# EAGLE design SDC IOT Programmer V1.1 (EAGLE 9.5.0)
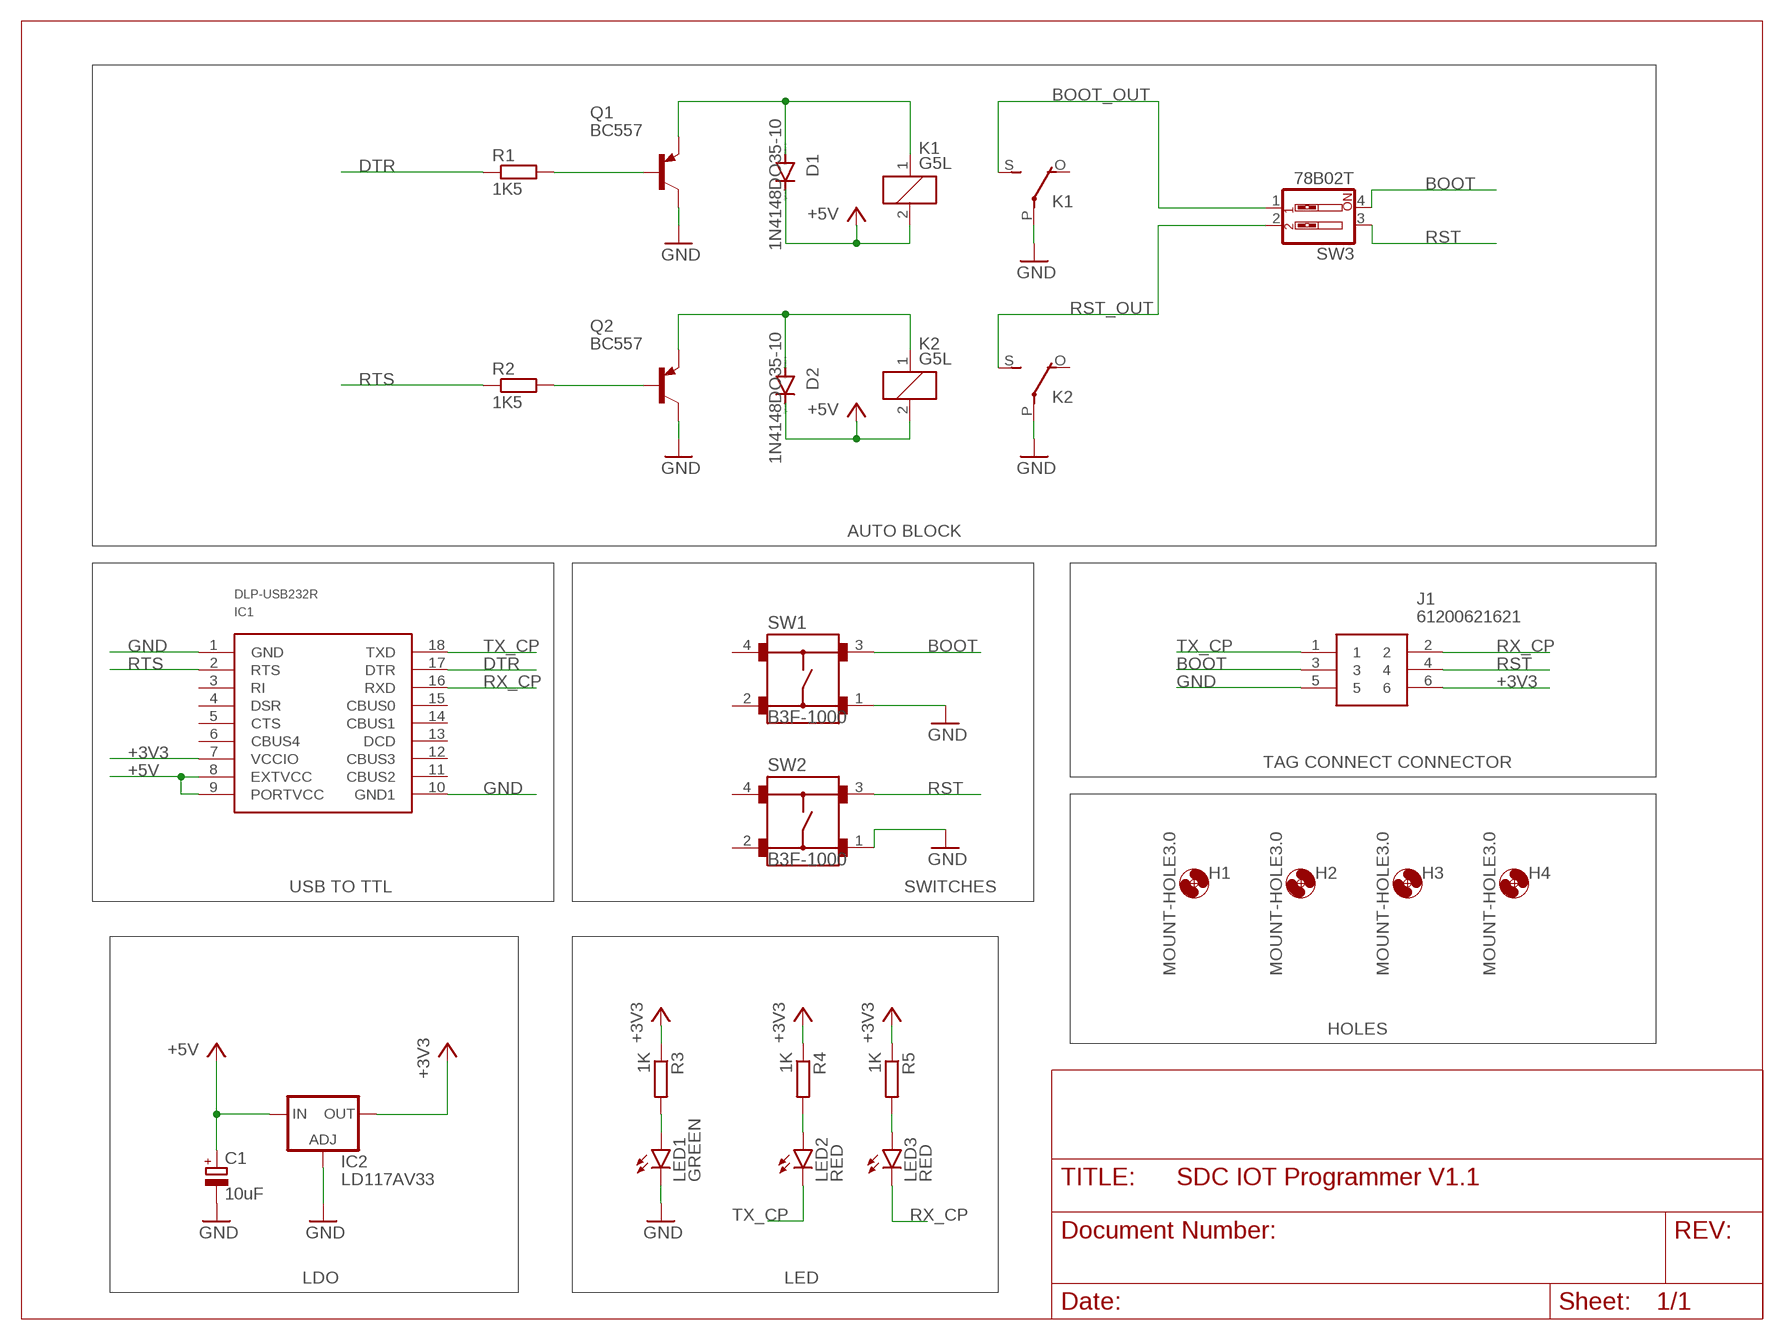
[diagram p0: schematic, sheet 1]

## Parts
C1  10uF  CPOL-EUE2.5-5  [E2,5-5]
D1  1N4148DO35-10  [DO35-10]
D2  1N4148DO35-10  [DO35-10]
H1  MOUNT-HOLE3.0  [3,0]
H2  MOUNT-HOLE3.0  [3,0]
H3  MOUNT-HOLE3.0  [3,0]
H4  MOUNT-HOLE3.0  [3,0]
IC1  DLP-USB232R  [DLP-USB232R]
IC2  LD117AV33  [TO220L1]
J1  61200621621  [SHDR6W64P254_2X3_1528X910X910P]
K1  G5L  [G5LE]
K2  G5L  [G5LE]
LED1  GREEN  LED3MM  [LED3MM]
LED2  RED  LED3MM  [LED3MM]
LED3  RED  LED3MM  [LED3MM]
Q1  BC557  [TO92-EBC]
Q2  BC557  [TO92-EBC]
R1  1K5  R-EU_0207/10  [0207/10]
R2  1K5  R-EU_0207/10  [0207/10]
R3  1K  R-EU_0207/10  [0207/10]
R4  1K  R-EU_0207/10  [0207/10]
R5  1K  R-EU_0207/10  [0207/10]
SW1  B3F-1000  [B3F-1000]
SW2  B3F-1000  [B3F-1000]
SW3  78B02T  SW_DIP-2  [EDG-02]

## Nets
+3V3: IC1.7(VCCIO) IC2.2(OUT) J1.6 R3.1 R4.1 R5.1
+5V: C1.+ D1.C D2.C IC1.8(EXTVCC) IC1.9(PORTVCC) IC2.3(IN) K1.2 K2.2
BOOT: J1.3 SW1.3 SW3.4
BOOT_OUT: K1.S(2:S) SW3.1
DTR: IC1.17(DTR) R1.1
GND: C1.- IC1.1(GND) IC1.10(GND1) IC2.1(ADJ) J1.5 K1.P(2:P) K2.P(2:P) LED1.K(C) Q1.C Q2.C SW1.1 SW2.1
N$7: LED2.A R4.2
N$12: Q1.B R1.2
N$13: Q2.B R2.2
N$14: D1.A K1.1 Q1.E
N$15: D2.A K2.1 Q2.E
N$16: LED1.A R3.2
N$17: LED3.A R5.2
RST: J1.4 SW2.3 SW3.3
RST_OUT: K2.S(2:S) SW3.2
RTS: IC1.2(RTS) R2.1
RX_CP: IC1.16(RXD) J1.2 LED3.K(C)
TX_CP: IC1.18(TXD) J1.1 LED2.K(C)
Unconnected: IC1.3(RI) IC1.4(DSR) IC1.5(CTS) IC1.6(CBUS4) IC1.11(CBUS2) IC1.12(CBUS3) IC1.13(DCD) IC1.14(CBUS1) IC1.15(CBUS0) K1.O(2:O) K2.O(2:O) SW1.2 SW1.4 SW2.2 SW2.4

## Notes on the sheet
- AUTO BLOCK
- TAG CONNECT CONNECTOR
- USB TO TTL | SWITCHES
- HOLES
- LDO | LED

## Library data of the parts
C1 = rcl:CPOL-EU: POLARIZED CAPACITOR, European symbol; SPICEPREFIX: C
D1 D2 = diode:1N4148: DIODE
H1-H4 = holes:MOUNT-HOLE: MOUNTING HOLE with drill center marker
IC1 = USB232:DLP-USB232R
IC2 = v-reg:LD117A?*: Low drop fixed and adjustable positive voltage regulators 1 A Source: http://www.st.com/stonline/products/literature/ds/7194/ld1117axx.pdf
J1 = MOLEX:61200621621: Wurth Elektronik PCB Header WR-BHD, 6 Way, 2.54mm Pitch, 2 Row, Straight, Through Hole Source: Datasheet; DESCRIPTION: Wurth Elektronik PCB Header WR-BHD, 6 Way, 2.54mm Pitch, 2 Row, Straight, Through Hole; HEIGHT: 9.1mm; MANUFACTURER_NAME: Wurth Elektronik; MANUFACTURER_PART_NUMBER: 61200621621; MOUSER_PART_NUMBER: 710-61200621621; MOUSER_PRICE-STOCK: https://www.mouser.co.uk/ProductDetail/Wurth-Elektronik/61200621621?qs=PhR8RmCirEbjX8n1RKw4Jw%3D%3D
K1 K2 = relay:G5L: RELAY 1 x switch, 10 A/120 V AC, 8 A/30 V ADC, Omron; OC_FARNELL: unknown; OC_NEWARK: unknown
LED1-LED3 = led:LED: LED
Q1 Q2 = transistor-pnp:BC557*: PNP Transistror
R1-R5 = rcl:R-EU_: RESISTOR, European symbol; SPICEPREFIX: R
SW1 SW2 = Switch:B3F-1000: Tactile Switch SPST-NO Top Actuated Through Hole Manufacturer's datasheet; CREATED_BY: PCBLayout.com; DIGI_KEY_PART_NUMBER: SW400-ND; MANUFACTURER: Omron Electronics Inc-EMC Div; MPN: B3F-1000; PACKAGE: SPST-NO
SW3 = special:SW_DIP-2: DIP SWITCH

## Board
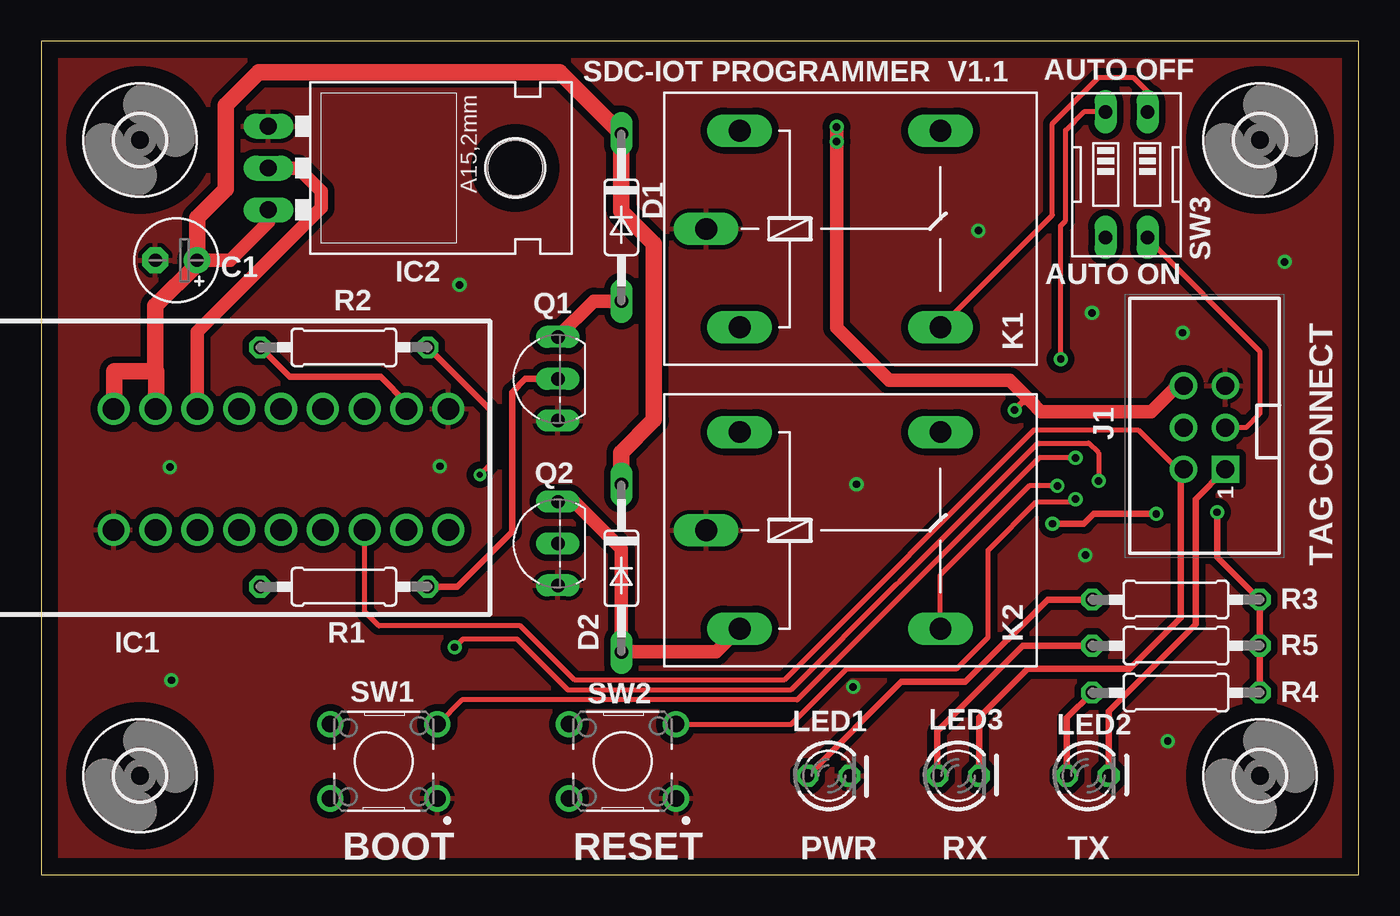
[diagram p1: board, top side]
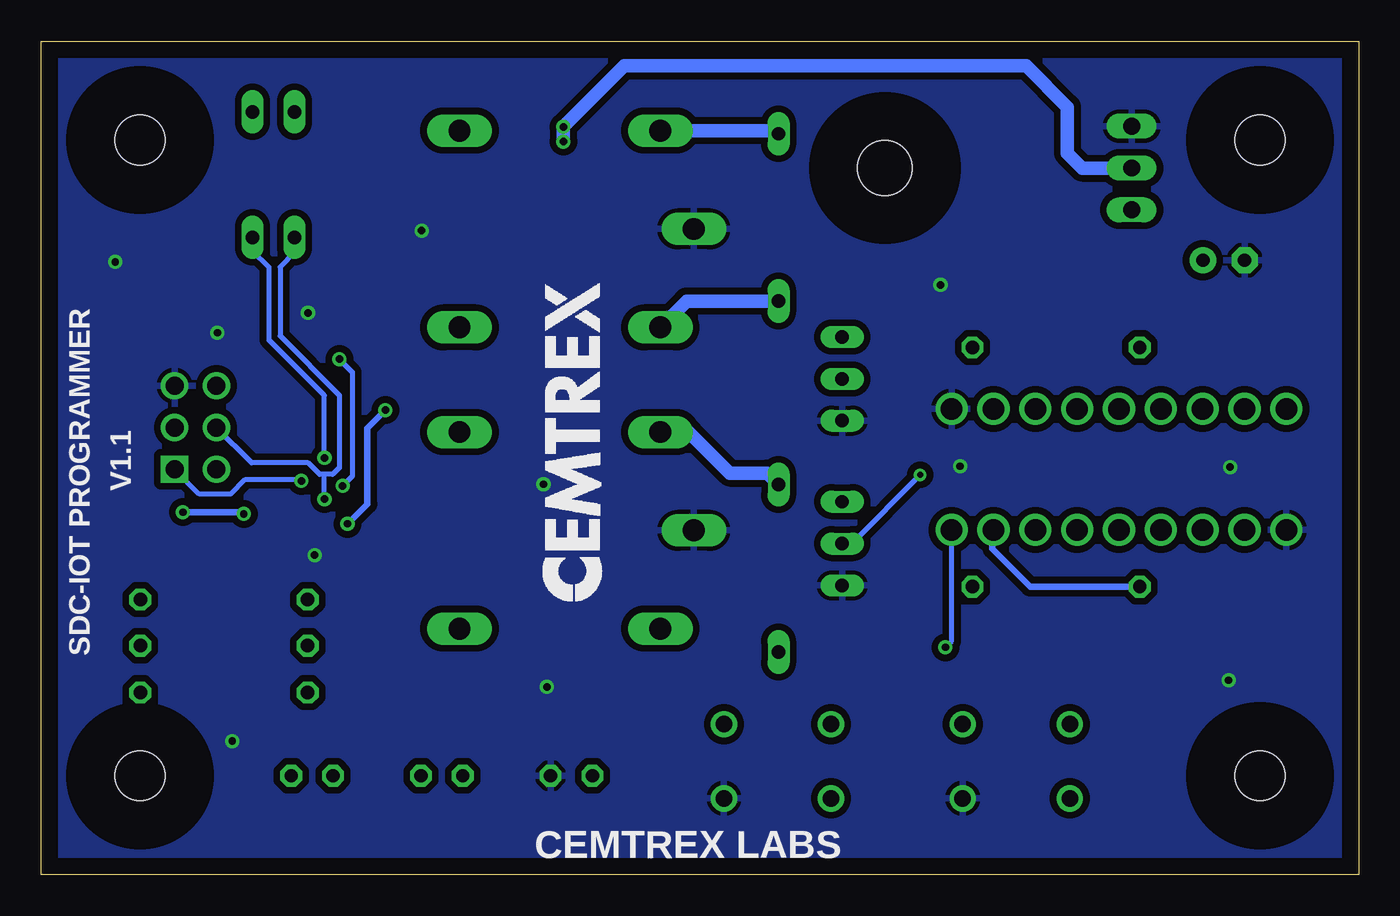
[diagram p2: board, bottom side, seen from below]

Size 80 x 50.6 mm. Coordinates in mm from the lower left corner, seen from the top.
Outline: 0,0 80,0 80,50.6 0,50.6 0,0
Copper layers (1*16): Top 0.035mm / dielectric 1.5mm / Bottom 0.035mm
Design rules "default *": minimum track width 8mil, minimum drill 0.35mm, track to track 6mil, track to pad 7mil, pad to pad 8mil, via to via 8mil, smd to smd 8mil, copper to edge 40mil, drill to drill 6mil, minimum pad ring 10mil, minimum via ring 8mil, stop-mask expansion 4mil, vias tented up to drill 20mil, thermal gap 10mil

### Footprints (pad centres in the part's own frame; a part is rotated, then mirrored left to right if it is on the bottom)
E2,5-5 = drill 0.813 pad 1.6: + -1.27,0 | drill 0.813 pad 1.6 octagon: - 1.27,0
DO35-10 = drill 0.813 long: A 5.08,0; C -5.08,0
3,0 = hole 3: 0,0
DLP-USB232R = drill 1.3: 1 -3.575,20.32; 2 -3.575,17.78; 3 -3.575,15.24; 4 -3.575,12.7; 5 -3.575,10.16; 6 -3.575,7.62; 7 -3.575,5.08; 8 -3.575,2.54; 9 -3.575,0; 10 3.77,0; 11 3.77,2.54; 12 3.77,5.08; 13 3.77,7.62; 14 3.77,10.16; 15 3.77,12.7; 16 3.77,15.24; 17 3.77,17.78; 18 3.77,20.32
TO220L1 = drill 1.016 long: 1 -2.54,-3.81; 2 0,-3.81; 3 2.54,-3.81 | hole 3.302: 0,11.176
SHDR6W64P254_2X3_1528X910X910P = drill 1.1 pad 1.65 square: 1 0,0 | drill 1.1 pad 1.65: 2 0,2.54; 3 2.54,0; 4 2.54,2.54; 5 5.08,0; 6 5.08,2.54
G5LE = drill 1.321 long: 1 -7.493,-5.969; 2 -7.493,5.969; O 4.699,5.969; P -9.525,0; S 4.699,-5.969
LED3MM = drill 0.813 octagon: A -1.27,0; K 1.27,0
TO92-EBC = drill 0.813 long: B 0,-1.27; C -2.54,-1.27; E 2.54,-1.27
0207/10 = drill 0.813 octagon: 1 -5.08,0; 2 5.08,0
B3F-1000 = drill 1 pad 1.6: 1 -3.25,2.25; 2 3.25,2.25; 3 -3.25,-2.25; 4 3.25,-2.25
EDG-02 = drill 0.813 long: 1 -1.27,-3.81; 2 1.27,-3.81; 3 1.27,3.81; 4 -1.27,3.81

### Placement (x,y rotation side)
C1  8.2,37.3 180 top
D1  35.22,39.9 270 top
D2  35.22,18.6 270 top
H1  6,6 0 top
H2  74,44.6 0 top
H3  74,6 0 top
H4  6,44.6 0 top
IC1  4.4,24.7 270 top
IC2  17.6,42.9 270 top
J1  71.9,24.6 90 top
K1  49.9,39.2 0 top
K2  49.9,20.9 0 top
LED1  47.8,6 0 top
LED2  63.55,6 0 top
LED3  55.67,6 0 top
Q1  30.1,30.1 90 top
Q2  30.1,20.1 90 top
R1  18.38,17.48 0 top
R2  18.38,32.01 0 top
R3  68.9,16.7 180 top
R4  68.9,11.05 180 top
R5  68.9,13.9 180 top
SW1  20.8,6.88 180 top
SW2  35.3,6.88 180 top
SW3  65.9,42.5 180 top

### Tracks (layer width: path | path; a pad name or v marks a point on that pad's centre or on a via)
+3V3  (via drill 0.45)
  Top 0.406: R4.1 R5.1 R3.1 71.4,19.28 v71.4,22 | v67.7,21.9 63.9,21.9 63.3,21.3 v61.4,21.3 | v59.1,28.2 59.6,28.7 60.1,28.7
  Top 0.813: J1.6 68.98,29.68 67.4,28.1 60.7,28.1 60.1,28.7 58.8,30 51.5,30 48.29,33.21 48.29,45.39 v48.3,45.4 | IC1.7 9.48,32.96 17,40.48 17,41.5 15.6,42.9 IC2.2
  Bottom 0.406: v71.4,22 67.8,22 v67.7,21.9 | v61.4,21.3 60.2,22.5 60.2,27.1 v59.1,28.2
  Bottom 0.813: IC2.2 16.8,42.9 17.7,43.8 17.7,46.6 20.2,49.1 44.6,49.1 v48.3,45.4 v48.3,44.5
+5V
  Top 0.813: 9.47,37.07 C1.+ 11.47,37.3 13.79,39.62 IC2.3
  Top 1.016: IC1.9 4.44,28.31 4.44,30.55 6.98,30.55 6.98,28.31 IC1.8 6.93,28.26 6.86,28.26 | D2.C 35.22,25.62 37.2,27.6 37.2,38.3 35.22,40.28 D1.C 31.49,48.71 13.21,48.71 11.2,46.7 11.2,41.6 9.47,39.87 C1.+ | 6.94,30.55 6.94,34.54 9.47,37.07
  Bottom 0.813: D1.C 35.41,45.17 K1.2 | D2.C 35.92,24.38 38.18,24.38 40.67,26.87 K2.2
BOOT  (via drill 0.45)
  Top 0.305: SW3.4 67.17,38.59 74,31.76 74,28 73.14,27.14 J1.3 | SW1.3 24.07,9.11 24.07,9.12 25.55,10.6 45.9,10.6 60.6,25.3 v62.8,25.3
  Bottom 0.305: v62.8,25.3 62.8,29.1 66.17,32.47 66.17,36.89 67.17,37.89 SW3.4
BOOT_OUT
  Top 0.305: K1.S 61.4,40.03 61.4,45.6 64.2,48.4 66.3,48.4 67.17,47.53 SW3.1
DTR
  Bottom 0.406: R1.1 19.96,17.48 22.25,19.77 22.25,20.86 IC1.17
GND  (via drill 0.45)
  other vias: 24.21,24.79 7.9,11.8 49.3,11.4 63.4,19.4 69.3,32.9 63.8,34.1 56.9,39.1 7.81,24.74 75.5,37.2 68.4,8.1 49.5,23.7 25.4,35.8
  pour Top (isolate 0.406): -0.8,51.4 -0.8,-0.6 81.4,-0.6 81.4,51.4
  pour Bottom (isolate 0.406): -0.7,51.3 -0.7,-0.7 81.2,-0.7 81.2,51.3
N$7
  Top 0.406: R4.2 62.28,9.51 LED2.A
N$12
  Top 0.406: Q1.B 29.4,30.1 28.6,29.3 28.6,20.81 25.27,17.48 R1.2
N$13  (via drill 0.35)
  Top 0.305: 27.19,28.27 27.19,24.83 v26.63,24.27
  Top 0.406: R2.2 27.19,28.27
  Bottom 0.305: v26.63,24.27 30.8,20.1 Q2.B
N$14
  Top 0.813: Q1.E 33.55,34.82 D1.A
  Bottom 0.813: D1.A 40.82,34.82 K1.1
N$15
  Top 0.813: K2.1 41,13.52 D2.A 35.22,19.78 32.36,22.64 Q2.E
N$16
  Top 0.406: R3.2 61.1,16.7 56.1,11.7 52.23,11.7 LED1.A
N$17
  Top 0.406: LED3.A 54.41,8.71 59.6,13.9 R5.2
RST  (via drill 0.45)
  Top 0.305: SW2.3 45.58,9.13 45.57,9.15 48.92,12.5 55.6,12.5 57.5,14.4 57.5,19.7 60.4,22.6 62.6,22.6 v62.8,22.8
  Bottom 0.305: J1.4 67.22,25 63.8,25 63.1,24.3 62.8,24.3 | SW3.3 64.63,37.77 65.5,36.9 65.5,32.7 61.9,29.1 61.9,24.7 62.3,24.3 62.8,24.3 | v62.8,22.8 62.8,24.3
RST_OUT  (via drill 0.45)
  Top 0.305: SW3.2 63.31,46.31 62.2,45.2 62.2,39.7 61.9,39.4 v61.9,31.3 | K2.S 54.6,18.2 60,23.6 v61.7,23.6
  Bottom 0.305: v61.9,31.3 61.1,30.5 61.1,24.2 v61.7,23.6
RTS
  Top 0.406: IC1.2 22.18,28.66 20.62,30.21 15.09,30.21 R2.1
RX_CP
  Top 0.305: 69.18,24.42 66.6,27 60.3,27 45.1,11.8 32.4,11.8 29.1,15.1 20.5,15.1 19.64,15.96 IC1.16
  Top 0.406: LED3.K 56.95,9.54 59.9,12.5 66.1,12.5 69.2,15.6 69.2,24.44 | 69.18,24.42 69.2,24.44 | 69.2,24.44 J1.2
TX_CP  (via drill 0.45)
  Top 0.305: v64.2,23.9 64.2,25.6 63.6,26.2 60.5,26.2 52.15,17.85 51.9,17.6 45.5,11.2 32,11.2 28.9,14.3 25.6,14.3 v25.1,13.8
  Top 0.406: LED2.K 64.82,9.92 70.1,15.2 70.1,22.8 J1.1
  Bottom 0.305: v64.2,23.9 64.3,24 67.6,24 68.5,23.1 70.4,23.1 J1.1 | v25.1,13.8 24.72,14.18 IC1.18

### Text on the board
tNames: AUTO OFF | SDC-IOT PROGRAMMER | V1.1 | AUTO ON | TAG CONNECT | 1 | BOOT | RESET | PWR | RX | TX
bNames: SDC-IOT PROGRAMMER | V1.1 | CEMTREX LABS
Measures: M3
